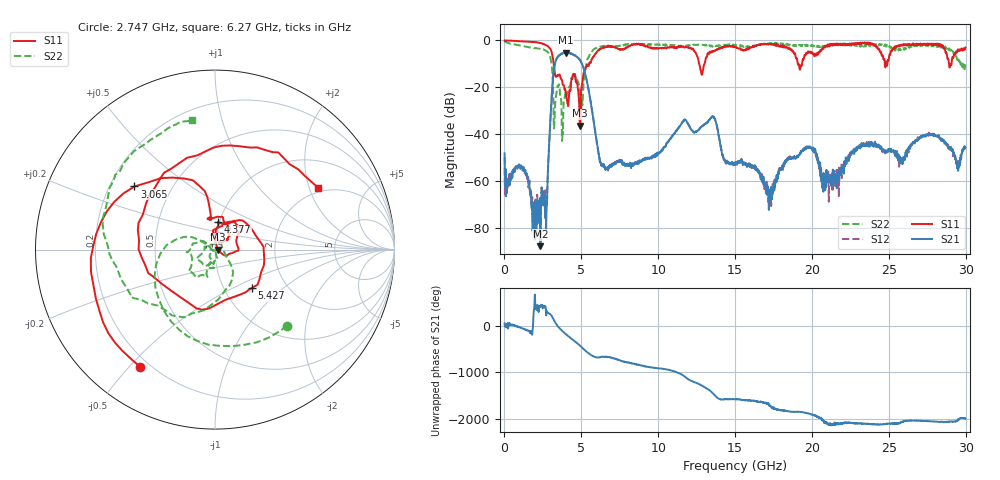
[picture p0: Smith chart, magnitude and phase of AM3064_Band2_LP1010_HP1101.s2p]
# Hz S DB R 50.0
!freq dBS11 angS11 dBS21 angS21 dBS12 angS12 dBS22 angS22
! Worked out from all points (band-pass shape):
!   1600 points, 10 MHz to 29.98 GHz, reference 50 ohm
!   highest |S21| = -5.24 dB at 3.984 GHz (marker M1); lowest = -87.8 dB at 2.334 GHz (marker M2)
!   |S21| within 3 dB of the highest: 3.368 GHz to 4.887 GHz (1.519 GHz wide, 36.8 % of centre)
!   lowest |S11| = -36.4 dB at 4.902 GHz (marker M3), VSWR 1.03, Z = 51.5 + j0.00864 ohm
!   |S11| at or under -10 dB: 3.204 GHz to 5.508 GHz (2.304 GHz wide, 52.9 % of centre); 12.66 GHz to 13 GHz (337.7 MHz wide, 2.63 % of centre); 19.08 GHz to 19.36 GHz (279.5 MHz wide, 1.45 % of centre)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
!   |S22| runs from -42.9 to -0.2 dB; largest |S21 - S12| = 0.017
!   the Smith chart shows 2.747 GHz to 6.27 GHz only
!   S11 on the Smith chart (normalised r, x): 2.747 GHz: 0.16, -0.54; 3.065 GHz: 0.30, +0.32; 4.377 GHz: 0.98, +0.31; 5.427 GHz: 1.34, -0.63; 6.27 GHz: 1.83, +2.30
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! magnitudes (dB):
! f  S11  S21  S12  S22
! 10 MHz  0.0  -48.2  -49.9  -0.2
! 1.36 GHz  -0.5  -56.4  -55.2  -2.7
! 1.959 GHz  -0.8  -68.9  -68.8  -3.3
! 2.334 GHz  -1.2  -87.8  -73.7  -3.6
! 2.747 GHz  -2.2  -71.2  -70.3  -4.7
! 3.065 GHz  -4.9  -24.8  -24.8  -10.3
! 3.346 GHz  -15.5  -8.4  -8.4  -23.8
! 3.984 GHz  -21.7  -5.2  -5.2  -22.0
! 4.377 GHz  -16.2  -5.8  -5.7  -16.1
! 4.902 GHz  -36.4  -8.4  -8.3  -21.3
! 5.015 GHz  -19.8  -9.7  -9.6  -26.5
! 5.427 GHz  -10.6  -19.7  -19.5  -7.6
! 6.27 GHz  -3.5  -52.4  -53.2  -2.7
! 10 GHz  -3.4  -48.2  -48.1  -1.8
! 12.83 GHz  -14.7  -36.7  -36.7  -1.9
! 13.54 GHz  -5.0  -32.6  -32.4  -2.6
! 15 GHz  -2.7  -52.4  -52.2  -1.9
! 17.25 GHz  -1.5  -63.8  -67.8  -1.2
! 19.99 GHz  -5.0  -46.2  -46.5  -1.9
! 20.78 GHz  -2.8  -61.2  -58.2  -3.0
! 25 GHz  -8.2  -47.2  -47.4  -2.2
! 29.98 GHz  -3.1  -45.8  -45.3  -10.2
